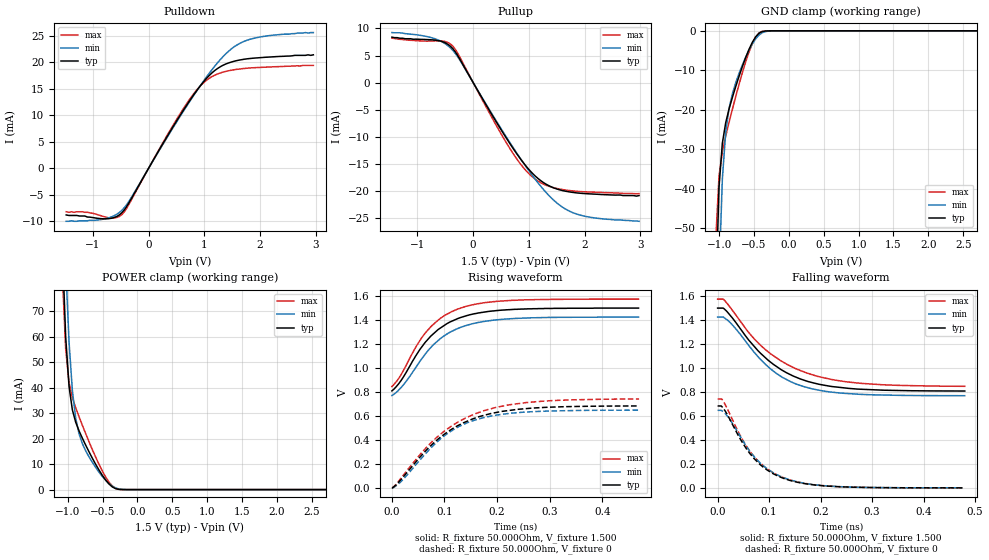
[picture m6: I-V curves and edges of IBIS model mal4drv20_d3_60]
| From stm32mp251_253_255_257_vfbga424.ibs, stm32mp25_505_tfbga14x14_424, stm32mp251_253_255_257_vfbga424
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[Model] mal4drv20_d3_60
Model_type   I/O
Polarity   Non-Inverting
Enable   Active-High
C_comp   1.836pF   1.830pF   1.844pF
C_comp_pullup   929.639fF   923.197fF   937.397fF
C_comp_pulldown 781.611fF   776.676fF   790.636fF
Vinh = 885.000mV
Vinl = 615.000mV
Vmeas = 750.000mV
Vref = 750.000mV
Rref = 50Ohms
Cref = 0pF
[Model Spec]
Vinh   885.000mV   848.000mV   923.000mV
Vinl   615.000mV   578.000mV   653.000mV
Vmeas   750.000mV   713.000mV   788.000mV
Vref   750.000mV   713.000mV   788.000mV
D_overshoot_ampl_h 0.4 NA   NA
D_overshoot_ampl_l 0.4 NA   NA
D_overshoot_area_l 100.000m NA   NA
D_overshoot_area_h 100.000m NA   NA
[Receiver Thresholds]
Vth = 750.000mV
Vth_min = 713.000mV
Vth_max = 788.000mV
Vinh_ac = 135.000mV
Vinh_dc = 100.000mV
Vinl_ac = -135.000mV
Vinl_dc = -100.000mV
Tslew_ac = 5.000ns
Threshold_sensitivity = 0.5
Reference_supply Pullup_ref
[Temperature Range]   25.000   125.000   -40.000
[Voltage Range]   1.500V   1.425V   1.575V
[GND Clamp Reference]   0.00V   0.00V   0.00V
[C Comp Corner]
| variable   typ   min   max
C_comp 1.844pF   1.836pF   1.830pF
C_comp_pullup 929.639fF   937.397fF   923.197fF
C_comp_pulldown 776.676fF   790.636fF   781.611fF
[Pulldown Reference]   0.00V   0.00V   0.00V
[POWER Clamp Reference]   1.500V   1.425V   1.575V
[Pullup Reference]   1.500V   1.425V   1.575V
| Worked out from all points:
|   slope of the pulldown table from 0 to 0.225 V, typ, clamps not added: 55.2 ohm
|   slope of the pullup table from 0 to 0.225 V, typ, clamps not added: 56.3 ohm
|   GND clamp passes 1 mA (typ) near -0.45 V on its own axis
|   POWER clamp passes 1 mA (typ) near -0.36 V on its own axis
|   rising waveform, R_fixture 50.000Ohm, V_fixture 1.500: 20-80 % time 76.3ps typ, 79.6ps min, 73.6ps max; typ from 0.808 V to 1.5 V
|   rising waveform, R_fixture 50.000Ohm, V_fixture 0: 20-80 % time 108ps typ, 97.4ps min, 116ps max; typ from -0.002 V to 0.682 V
|   falling waveform, R_fixture 50.000Ohm, V_fixture 1.500: 20-80 % time 102ps typ, 93.6ps min, 115ps max; typ from 1.5 V to 0.809 V
|   falling waveform, R_fixture 50.000Ohm, V_fixture 0: 20-80 % time 73.9ps typ, 75.2ps min, 73.5ps max; typ from 0.684 V to 0 V
[GND Clamp]
-1.48V    -1.637A    -1.644A    -1.658A
-1.05V    -67.86mA   -111.2mA   -53.06mA
-1.002V   -39.45mA   -62.21mA   -36.77mA
-954.6mV  -28.48mA   -37.5mA    -30.67mA
-906.8mV  -23.32mA   -25.75mA   -26.73mA
-859.1mV  -19.86mA   -19.72mA   -23.25mA
-763.6mV  -14.17mA   -13.2mA    -16.7mA
-668.2mV  -9.09mA    -8.668mA   -10.65mA
-525mV    -2.932mA   -3.341mA   -3.236mA
-429.5mV  -625.7uA   -1.091mA   -535.7uA
-238.6mV  -2.309uA   -20.7uA    -473nA
2.959V    72.19nA    968.6nA    105nA
[Power Clamp]
-1.459V   654.6mA    675.2mA    655.4mA
-1.077V   94.79mA    129.9mA    83.6mA
-1.03V    59.92mA    88.13mA    55.16mA
-981.8mV  40.46mA    57.96mA    42.01mA
-934.1mV  31.26mA    38.88mA    36.03mA
-886.4mV  26.43mA    28.01mA    32.07mA
-838.6mV  23.06mA    21.89mA    28.58mA
-647.7mV  12.32mA    10.7mA     15.7mA
-504.6mV  5.603mA    5.163mA    7.311mA
-361.4mV  1.062mA    1.366mA    1.412mA
-218.2mV  16.86uA    87.94uA    13.19uA
2.98V     -71.2nA    -1.524uA   -71.42nA
[Pulldown]
-1.48V    -8.8mA     -10mA      -8.2mA
-1.098V   -9.2mA     -9.9mA     -8.3mA
-763.6mV  -9.53mA    -9.49mA    -9.24mA
-477.3mV  -8.362mA   -7.898mA   -8.711mA
-334.1mV  -6.179mA   -5.928mA   -6.443mA
286.4mV   5.17mA     5.029mA    5.361mA
668.2mV   11.65mA    11.47mA    11.94mA
906.8mV   15.25mA    15.24mA    15.29mA
1.145V    18.06mA    18.69mA    17.34mA
1.48V     20.02mA    22.46mA    18.48mA
1.766V    20.64mA    24.14mA    18.88mA
2.959V    21.4mA     25.6mA     19.4mA
[Pullup]
-1.459V   8.4mA      9.243mA    8.2mA
-743.2mV  7.9mA      8.28mA     7.679mA
-504.6mV  7.367mA    7.204mA    7.597mA
-361.4mV  6.232mA    5.912mA    6.694mA
-265.9mV  4.802mA    4.583mA    5.225mA
688.6mV   -11.74mA   -11.55mA   -12.66mA
927.3mV   -15.16mA   -15.23mA   -16.03mA
1.166V    -17.75mA   -18.56mA   -18.22mA
1.5V      -19.67mA   -22.23mA   -19.59mA
1.786V    -20.31mA   -24.05mA   -20.04mA
2.168V    -20.63mA   -25.02mA   -20.27mA
2.98V     -20.9mA    -25.66mA   -20.54mA
[Ramp]
R_load=50.000Ohm
dV/dt_r   412.320mV/93.000ps  390.807mV/89.500ps  440.820mV/96.000ps
dV/dt_f   412.320mV/89.000ps  390.808mV/85.500ps  440.820mV/95.500ps
[Rising waveform]
R_fixture=50.000Ohm
V_fixture=1.500
V_fixture_min=1.425
V_fixture_max=1.575
0s        807.9mV    769.5mV    844.4mV
12ps      862.7mV    810.8mV    906.3mV
24ps      939.3mV    869.9mV    995.3mV
49ps      1.126V     1.027V     1.201V
67ps      1.233V     1.135V     1.311V
95ps      1.343V     1.255V     1.423V
125ps     1.412V     1.329V     1.492V
174ps     1.466V     1.388V     1.544V
231ps     1.489V     1.413V     1.565V
469ps     1.5V       1.425V     1.575V
[Rising waveform]
R_fixture=50.000Ohm
V_fixture=0
0s        -2.483mV   -1.455mV   -2.376mV
6ps       14.43mV    8.508mV    18.23mV
18ps      70.37mV    52.75mV    82.16mV
58ps      277.7mV    253.8mV    298.7mV
84ps      390.7mV    374mV      414.8mV
117ps     496.7mV    484.8mV    524.8mV
159ps     582.4mV    565.8mV    617.8mV
220ps     643.2mV    618.3mV    689.9mV
275ps     666.2mV    636.2mV    718.7mV
470ps     682.2mV    647mV      740.4mV
[Falling waveform]
R_fixture=50.000Ohm
V_fixture=1.500
V_fixture_min=1.425
V_fixture_max=1.575
0s        1.502V     1.427V     1.577V
11ps      1.502V     1.427V     1.577V
24ps      1.444V     1.383V     1.511V
65ps      1.211V     1.165V     1.274V
92ps      1.09V      1.036V     1.158V
126ps     981.1mV    923mV      1.054V
174ps     890.6mV    838.1mV    958.8mV
216ps     850.5mV    802.6mV    909.6mV
272ps     825.2mV    782.4mV    875.3mV
480ps     809.1mV    770.1mV    848.6mV
[Falling waveform]
R_fixture=50.000Ohm
V_fixture=0
0s        684.3mV    647.9mV    742.2mV
11ps      665.1mV    635.8mV    723.9mV
24ps      570.7mV    570.2mV    614.5mV
47ps      385.9mV    406.5mV    412.5mV
72ps      239.6mV    255.4mV    255.4mV
96ps      149.8mV    160.5mV    159.1mV
128ps     79.32mV    84.94mV    84.25mV
170ps     34.6mV     36.95mV    37.08mV
227ps     11.13mV    12.19mV    11.51mV
476ps     59.61uV    88.42uV    63.39uV
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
